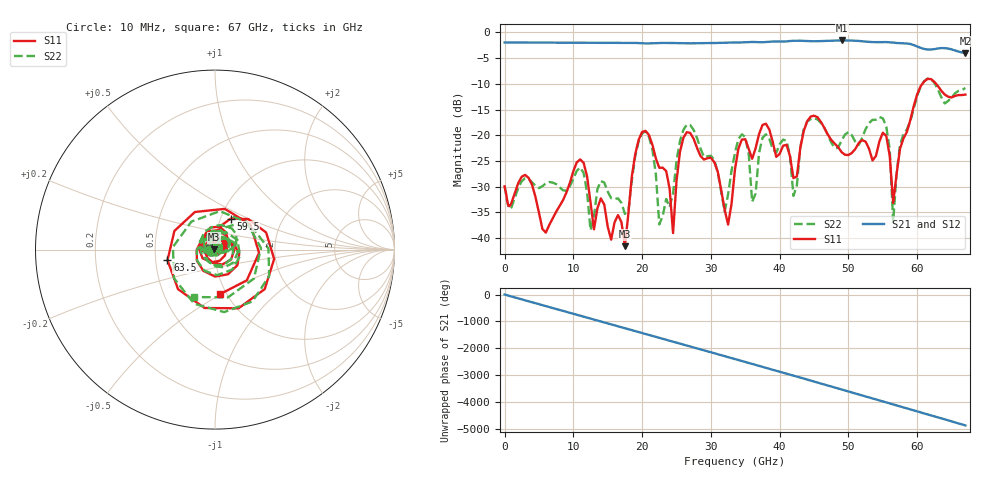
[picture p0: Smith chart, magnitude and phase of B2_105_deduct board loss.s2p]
!Keysight Technologies,N5247B,MY61255065,A.16.20.04
!Date: Sunday, September 03, 2023 22:02:55
!Correction: S11(C  2-Port  )
!S21(C  2-Port  )
!S12(C  2-Port  )
!S22(C  2-Port  )
!S2P File: Measurements: S11, S21, S12, S22:
!Deduct Board Loss
# Hz S  dB  R 50
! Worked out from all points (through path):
!   142 points, 10 MHz to 67 GHz, reference 50 ohm
!   highest |S21| = -1.55 dB at 49 GHz (marker M1); lowest = -4.0 dB at 67 GHz (marker M2)
!   lowest |S11| = -41.6 dB at 17.5 GHz (marker M3), VSWR 1.02, Z = 49.2 + j0.189 ohm
!   |S11| at or under -10 dB: start of sweep to 60.74 GHz; 62.74 GHz to end of sweep
!   |S22| runs from -38.5 to -9.0 dB; largest |S21 - S12| = 0.0024
!   S11 on the Smith chart (normalised r, x): 10 MHz: 0.94, -0.00; 59.5 GHz: 1.12, +0.40; 63.5 GHz: 0.58, -0.07; 67 GHz: 0.94, -0.49
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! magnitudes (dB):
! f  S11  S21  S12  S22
! 10 MHz  -29.9  -2.0  -1.9  -29.9
! 6 GHz  -38.9  -2.0  -2.0  -29.3
! 11.5 GHz  -25.3  -2.0  -2.0  -27.4
! 12.5 GHz  -33.0  -2.0  -2.0  -38.5
! 14 GHz  -32.3  -2.0  -2.0  -28.9
! 17.5 GHz  -41.6  -2.0  -2.0  -35.3
! 20.5 GHz  -19.1  -2.1  -2.1  -19.3
! 22.5 GHz  -26.3  -2.0  -2.0  -37.3
! 24.5 GHz  -39.0  -2.0  -2.0  -31.4
! 26.5 GHz  -19.4  -2.1  -2.1  -17.9
! 32.5 GHz  -37.4  -2.0  -2.0  -31.5
! 34 GHz  -22.6  -2.0  -1.9  -20.7
! 36 GHz  -24.6  -1.8  -1.8  -32.9
! 38 GHz  -17.7  -1.9  -1.9  -19.8
! 42 GHz  -28.3  -1.6  -1.6  -31.8
! 45 GHz  -16.2  -1.7  -1.7  -16.7
! 49 GHz  -23.3  -1.5  -1.5  -21.0
! 56 GHz  -24.0  -1.9  -1.9  -22.7
! 56.5 GHz  -33.1  -2.0  -2.0  -36.8
! 59.5 GHz  -14.3  -2.5  -2.4  -14.7
! 63.5 GHz  -11.3  -3.0  -3.0  -12.6
! 67 GHz  -12.1  -4.0  -4.0  -10.8
